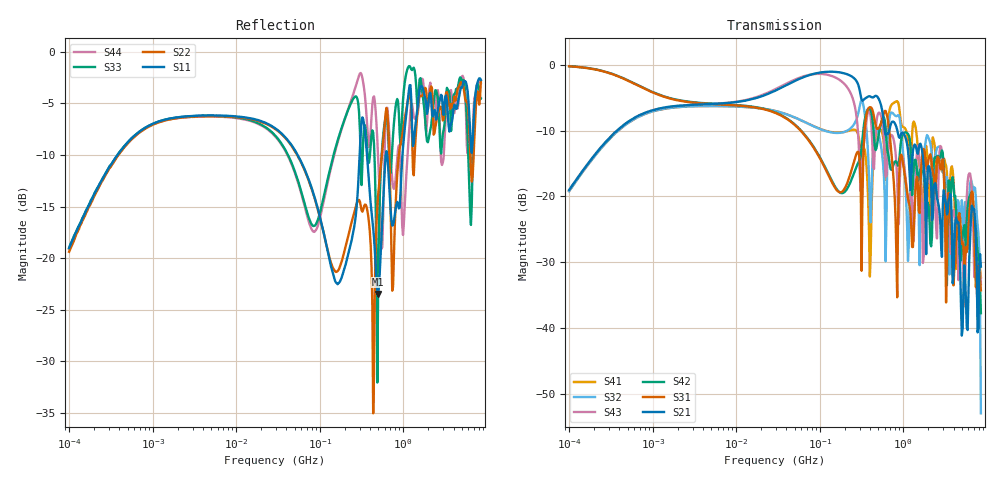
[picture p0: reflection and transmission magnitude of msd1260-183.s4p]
# MHz S MA R 50
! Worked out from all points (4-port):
!   498 points, 100 kHz to 8.5 GHz, reference 50 ohm
!   strongest paths, dB at 100 kHz, 1.698 MHz, 29.49 MHz, 500.7 MHz, 8.5 GHz:
!     S21: -19.0, -6.3, -3.9, -5.0, -30.6
!     S31: -0.3, -5.2, -7.3, -9.7, -34.2
!     S42: -0.2, -5.2, -7.3, -11.1, -37.7
!     S43: -19.0, -6.4, -3.7, -7.4, -33.3
!     S32: -19.2, -6.5, -7.0, -10.2, -52.9
!     S41: -19.2, -6.5, -7.0, -9.9, -32.2
!   lowest |S11| = -23.5 dB at 500.7 MHz (marker M1), VSWR 1.14, Z = 55.6 - j4.35 ohm
!   |S11| at or under -10 dB: 54.48 MHz to 300.5 MHz (246 MHz wide, 139 % of centre); 368.2 MHz to 617.8 MHz (249.6 MHz wide, 50.6 % of centre); 641.8 MHz to 978.7 MHz (337 MHz wide, 41.6 % of centre)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
0.1  0.1123 75.4  0.112 75.8  0.9714 -6.5  0.1097 -104.8
     0.112 75.8  0.1075 75.8  0.1098 -104.6  0.9737 -6.4
     0.9714 -6.5  0.1098 -104.6  0.1119 75.5  0.1119 75.6
     0.1097 -104.8  0.9737 -6.4  0.1119 75.6  0.1104 75.8
500.661  0.0671 -35.5  0.5602 -96.9  0.3263 -35.1  0.321 -1.3
         0.5602 -96.9  0.2018 23.3  0.3082 -54.4  0.2792 -12.3
         0.3263 -35.1  0.3082 -54.4  0.07248 36.0  0.4263 -79.6
         0.321 -1.3  0.2792 -12.3  0.4263 -79.6  0.3074 -115.3
1139.211  0.5939 -89.6  0.2245 -169.8  0.09729 -168.8  0.2726 -144.0
          0.2245 -169.8  0.5871 -103.5  0.03248 87.4  0.298 -135.0
          0.09729 -168.8  0.03248 87.4  0.8385 -107.2  0.09466 -142.2
          0.2726 -144.0  0.298 -135.0  0.09466 -142.2  0.3407 -82.1
3257.229  0.6148 50.4  0.08588 -19.5  0.01571 -23.8  0.1709 -2.0
          0.08588 -19.5  0.6329 58.0  0.1325 -10.5  0.04278 -34.5
          0.01571 -23.8  0.1325 -10.5  0.6237 62.7  0.07948 29.4
          0.1709 -2.0  0.04278 -34.5  0.07948 29.4  0.5309 75.9
5142.985  0.6882 -92.1  0.01005 101.3  0.04463 -133.5  0.05484 -116.5
          0.01005 101.3  0.6964 -101.4  0.08023 -126.4  0.05023 -79.7
          0.04463 -133.5  0.08023 -126.4  0.7078 -101.1  0.04339 68.1
          0.05484 -116.5  0.05023 -79.7  0.04339 68.1  0.7653 -98.0
6920.76  0.4425 38.3  0.07975 -6.3  0.08659 16.2  0.0737 42.6
         0.07975 -6.3  0.2945 35.8  0.1112 50.3  0.08002 21.6
         0.08659 16.2  0.1112 50.3  0.4097 35.9  0.05162 -112.6
         0.0737 42.6  0.08002 21.6  0.05162 -112.6  0.5003 53.9
8500  0.7306 -53.3  0.02939 -102.6  0.01943 -102.8  0.02441 -128.3
      0.02939 -102.6  0.723 -38.4  0.002268 -114.2  0.01304 -123.2
      0.01943 -102.8  0.002268 -114.2  0.5941 -44.4  0.02169 -24.9
      0.02441 -128.3  0.01304 -123.2  0.02169 -24.9  0.7083 -55.2
